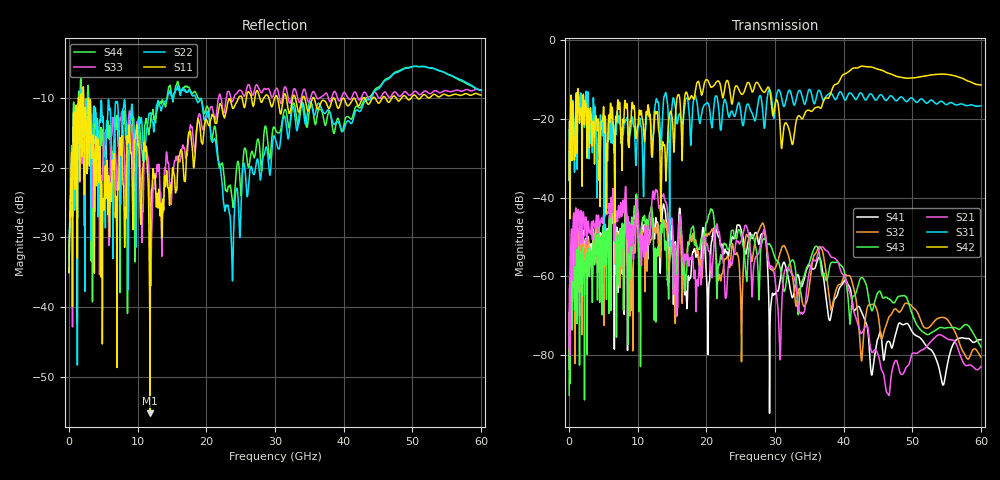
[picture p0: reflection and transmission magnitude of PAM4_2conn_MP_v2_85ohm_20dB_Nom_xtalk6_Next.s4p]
! Info: Touchstone file created by Circ.  Input file=FAB50GbE_2conn_Midplane_Examax_Topo2_v2_85ohm_20dB_Nom.circ
# Hz S RI R 50
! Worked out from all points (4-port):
!   6000 points, 10 MHz to 60 GHz, reference 50 ohm
!   strongest paths, dB at 10 MHz, 15.01 GHz, 30.01 GHz, 45.01 GHz, 60 GHz:
!     S42: -35.6, -19.6, -16.3, -7.5, -11.4
!     S31: -35.7, -16.6, -17.2, -14.7, -16.7
!     S21: -78.2, -45.5, -60.7, -79.7, -82.9
!     S43: -90.1, -52.4, -55.3, -64.1, -77.9
!     S32: -78.9, -51.8, -58.0, -69.7, -80.5
!     S41: -83.5, -46.3, -64.5, -75.8, -76.1
!   lowest |S11| = -55.3 dB at 11.8 GHz (marker M1), VSWR 1.00, Z = 50.2 - j0.0184 ohm
!   |S11| at or under -10 dB: 2.838 GHz to 24.67 GHz (21.84 GHz wide, 159 % of centre); 35.71 GHz to 38.47 GHz (2.763 GHz wide, 7.45 % of centre); 40.03 GHz to 41.42 GHz (1.385 GHz wide, 3.4 % of centre)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
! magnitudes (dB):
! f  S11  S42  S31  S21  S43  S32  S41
! 10 MHz  -35.1  -35.6  -35.7  -78.2  -90.1  -78.9  -83.5
! 1.19 GHz  -31.3  -27.6  -32.8  -52.9  -58.8  -59.6  -56.8
! 11.8 GHz  -55.3  -19.0  -19.1  -49.6  -43.8  -51.2  -48.8
! 23.76 GHz  -11.3  -16.3  -18.1  -56.7  -48.3  -51.9  -50.0
! 37.01 GHz  -10.3  -15.8  -15.3  -52.6  -59.5  -54.2  -59.5
! 44.1 GHz  -10.2  -6.9  -13.8  -79.1  -68.7  -67.1  -85.0
! 60 GHz  -9.5  -11.4  -16.7  -82.9  -77.9  -80.5  -76.1
